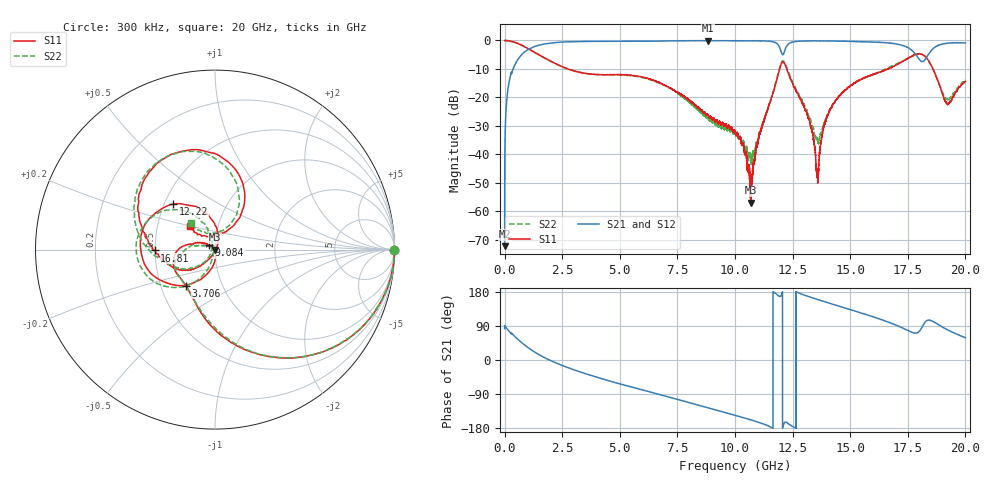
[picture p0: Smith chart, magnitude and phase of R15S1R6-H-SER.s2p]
!{R15S1R6}
!Johanson Technology Inc.
!www.johansontechnology.com
!Test Board Conditions:
!Substrate Type  RO4350B
!Substrate Thickness  20 mil
!Substrate Dk  3.66
!TL Type: GCPW
!TL Trace Width  34 mil
!TL Gap  10 mil
!Electrode orientation  Horizontal
!DUT TOPOLOGY	SERIES
!Mounting Pad LxW  26x52 mil
! Created Sat Feb  6 12:16:26 2021
# hz S ma R 50
! 2 Port Network Data from SP1.SP block
! freq  magS11  angS11  magS21  angS21  magS12  angS12  magS22  angS22
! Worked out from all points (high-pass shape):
!   20001 points, 300 kHz to 20 GHz, reference 50 ohm
!   highest |S21| = -0.06 dB at 8.841 GHz (marker M1); lowest = -72.2 dB at 300 kHz (marker M2)
!   |S21| within 3 dB of the highest: 1.048 GHz to 11.97 GHz (10.92 GHz wide, 168 % of centre); 12.18 GHz to 17.61 GHz (5.428 GHz wide, 36.4 % of centre)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
!   lowest |S11| = -57.0 dB at 10.68 GHz (marker M3), VSWR 1.00, Z = 49.9 - j0.0497 ohm
!   |S11| at or under -10 dB: 2.744 GHz to 11.94 GHz (9.194 GHz wide, 125 % of centre); 12.25 GHz to 16.63 GHz (4.381 GHz wide, 30.3 % of centre); 18.59 GHz to end of sweep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
!   |S22| runs from -43.5 to 0.0 dB; largest |S21 - S12| = 0.017
!   S11 on the Smith chart (normalised r, x): 300 kHz: open; 3.706 GHz: 0.67, -0.29; 9.084 GHz: 0.93, +0.05; 12.22 GHz: 0.56, +0.32; 16.81 GHz: 0.50, -0.01; 20 GHz: 0.73, +0.20
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300000  0.9953 0.0  0.0002442 82.7  0.0002544 98.1  0.9951 -0.2
1.313e8  0.9911 -9.1  0.1272 80.6  0.1277 80.6  0.9912 -9.1
4.983e8  0.9094 -30.8  0.4112 59.0  0.4122 59.0  0.9088 -30.7
1.7043e9  0.5011 -83.1  0.8611 7.3  0.8628 7.2  0.5003 -82.0
3.3343e9  0.2716 -122.3  0.9587 -32.6  0.9598 -32.6  0.2724 -122.1
3.7063e9  0.2579 -129.1  0.9628 -39.9  0.9636 -39.9  0.2583 -130.0
6.6673e9  0.185 175.0  0.9749 -90.1  0.9752 -90.1  0.1813 -175.5
8.8413e9  0.04781 144.6  0.9935 -126.4  0.9906 -126.4  0.04258 152.9
9.0843e9  0.04247 142.0  0.9919 -130.5  0.9928 -130.5  0.03714 148.0
1.00003e10  0.02518 141.5  0.9909 -145.9  0.9904 -145.9  0.02422 128.1
1.06793e10  0.001413 -159.3  0.9875 -157.8  0.9862 -157.8  0.008198 -170.4
1.18943e10  0.2728 -132.6  0.8144 169.1  0.8154 169.2  0.2864 -132.8
1.22163e10  0.3441 132.5  0.756 -164.1  0.7563 -164.4  0.3597 143.2
1.33343e10  0.02687 60.0  0.9819 164.6  0.9813 164.6  0.03136 118.5
1.35873e10  0.003915 -43.1  0.984 159.6  0.982 159.6  0.01763 175.0
1.38833e10  0.03353 -117.0  0.9826 153.9  0.9798 154.0  0.03651 -134.8
1.43223e10  0.08186 -126.8  0.9759 145.7  0.9776 145.7  0.08186 -129.4
1.66673e10  0.3172 -175.2  0.9063 99.7  0.8911 99.6  0.3327 -173.7
1.68113e10  0.3362 -179.2  0.8894 96.3  0.8801 96.4  0.356 -177.5
1.81073e10  0.5728 103.5  0.4254 85.4  0.4258 85.9  0.5748 108.2
1.91943e10  0.07857 91.8  0.8903 80.6  0.8913 80.7  0.09293 90.9
2e10  0.1898 137.0  0.904 58.7  0.8999 58.6  0.2028 131.9
